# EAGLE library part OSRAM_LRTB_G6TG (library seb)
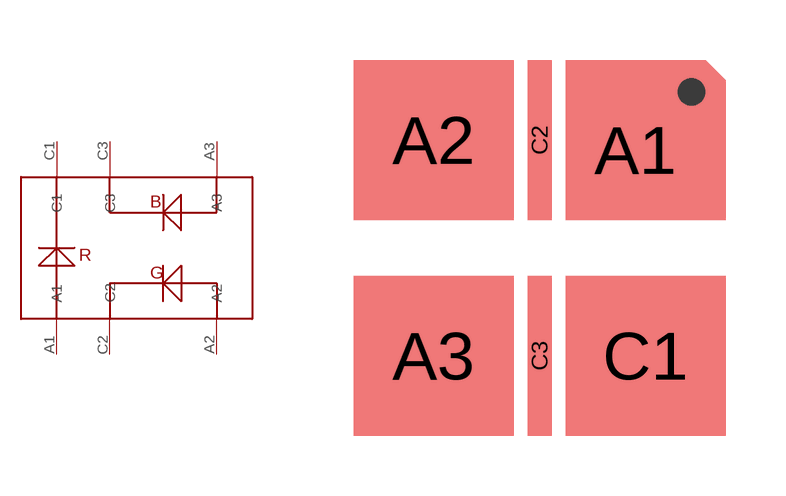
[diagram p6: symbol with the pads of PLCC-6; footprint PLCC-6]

Designator prefix D

## OSRAM_LRTB_G6TG  [PLCC-6]
A1  A1
A2  A2
A3  A3
C1  C1
C2  C2
C3  C3

## Footprint PLCC-6 (pad centres in mm)
smd 3.5 x 3.5: A1 2.4,2.45
smd 4 x 4: A2 -2.65,2.7; A3 -2.65,-2.7; C1 2.65,-2.7
smd 0.6 x 4: C2 0,2.7; C3 0,-2.7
